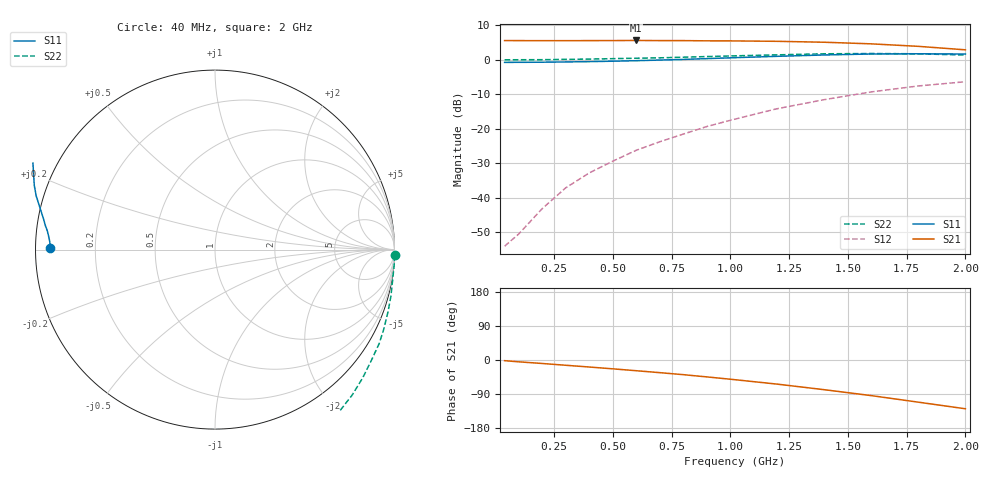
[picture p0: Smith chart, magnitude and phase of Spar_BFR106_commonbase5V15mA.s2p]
! Filename:  BFR106CA.S2P  Version:  2.0
! NXP part #: BFR106  Date: Jul 1990
! Bias condition: Vce=5V, Ic=15mA
! COMMON BASE
#  MHz  S  MA  R  50
! Freq  S11  S21  S12  S22
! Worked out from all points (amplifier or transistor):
!   16 points, 40 MHz to 2 GHz, reference 50 ohm
!   highest |S21| = 5.6 dB at 600 MHz (marker M1)
!   |S21| within 3 dB of that: start of sweep to end of sweep
!   unconditionally stable (mu >= 1): nowhere
!   at 200 MHz: K = -0.56, MSG = 24.3 dB, |S12| = -43.1 dB
!   at 800 MHz: K = -0.91, MSG = 13.5 dB, |S12| = -21.5 dB
!   at 2 GHz: K = -0.69, MSG = 4.6 dB, |S12| = -6.4 dB
40  0.918 179.6  1.898 -1.8  0.002 50.7  1.001 -1.8
100  0.919 178.3  1.896 -4.8  0.003 111.7  1.002 -4.9
200  0.923 176.9  1.892 -9.2  0.007 120.4  1.004 -9.7
300  0.931 175.2  1.893 -13.9  0.014 132.1  1.014 -14.8
400  0.941 173.5  1.896 -18.5  0.023 137.3  1.024 -19.7
500  0.954 172.0  1.898 -23.3  0.034 137.5  1.039 -25.0
600  0.971 169.8  1.906 -28.3  0.049 138.6  1.054 -29.8
700  0.991 167.7  1.896 -33.4  0.065 139.0  1.068 -35.4
800  1.013 165.6  1.896 -38.7  0.084 139.4  1.09 -41.0
900  1.04 163.3  1.882 -44.6  0.108 137.1  1.114 -46.7
1000  1.068 160.5  1.879 -50.7  0.133 134.6  1.138 -52.6
1200  1.123 154.6  1.852 -63.7  0.196 128.5  1.18 -65.1
1400  1.175 147.3  1.796 -78.4  0.265 120.8  1.222 -78.5
1600  1.214 139.2  1.702 -94.0  0.343 112.5  1.233 -92.6
1800  1.222 130.5  1.566 -111.3  0.418 102.7  1.222 -107.2
2000  1.213 122.7  1.395 -128.7  0.481 93.6  1.17 -122.0
